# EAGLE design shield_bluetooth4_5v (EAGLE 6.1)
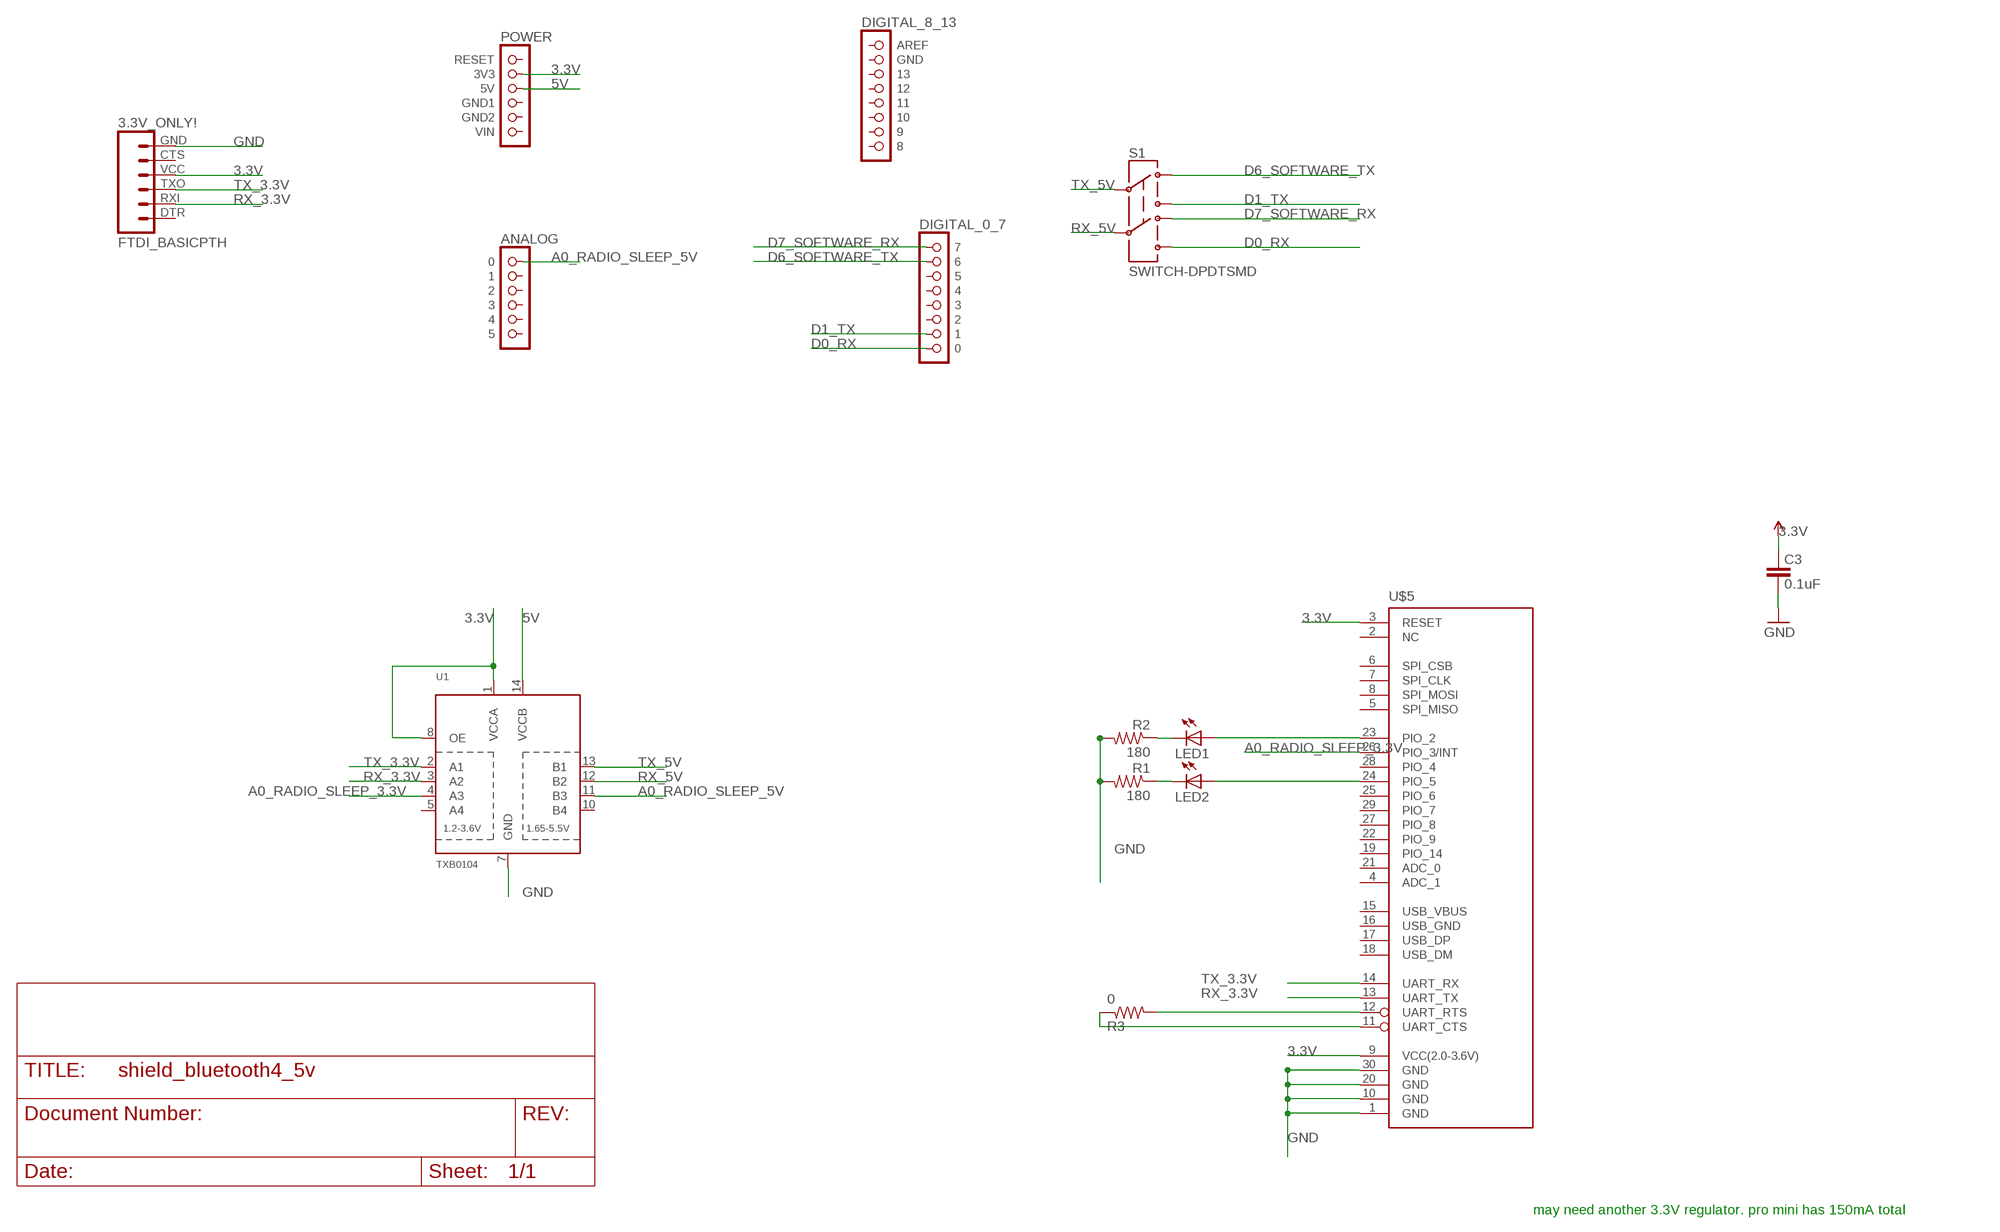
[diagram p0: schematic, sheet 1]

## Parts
3.3V_ONLY!  FTDI_BASICPTH  [FTDI_BASIC]
C3  0.1uF  CAP0402-CAP  [0402-CAP]
LED1  LED0603  [LED-0603]
LED2  LED0603  [LED-0603]
R1  180  RESISTOR0402-RES  [0402-RES]
R2  180  RESISTOR0402-RES  [0402-RES]
R3  0  RESISTOR0402-RES  [0402-RES]
S1  SWITCH-DPDTSMD  [AYZ0202]
U1  TXB0104  TXB0104PWRSOIC14  [SO14]
U$1  POWER  [1X06]
U$2  ANALOG  [1X06]
U$3  DIGITAL_0_7  [1X08]
U$4  DIGITAL_8_13  [1X08]
U$5  BLUERADIO_BR-LE4.0-S2  [BLUERADIO_BR-LE4.0-S2]

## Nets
3.3V: 3.3V_ONLY!.VCC C3.2 U1.1(VCCA) U1.8(OE) U$1.2(3V3) U$5.3(RESET) U$5.9(VCC(2.0-3.6V)) ; supply symbol labelled VCC
5V: U1.14(VCCB) U$1.3(5V)
A0_RADIO_SLEEP_3.3V: U1.4(A3) U$5.26(PIO_3/INT)
A0_RADIO_SLEEP_5V: U1.11(B3) U$2.1
D0_RX: S1.6 U$3.8
D1_TX: S1.3 U$3.7
D6_SOFTWARE_TX: S1.1 U$3.2
D7_SOFTWARE_RX: S1.4 U$3.1
GND [vcc]: 3.3V_ONLY!.GND C3.1 R1.2 R2.2 U1.7(GND) U$5.1(GND) U$5.10(GND) U$5.20(GND) U$5.30(GND)
N$1: LED2.A U$5.24(PIO_5)
N$2: LED1.C R2.1
N$3: LED1.A U$5.23(PIO_2)
N$4: LED2.C R1.1
N$5: R3.2 U$5.12(UART_RTS)
N$9: R3.1 U$5.11(UART_CTS)
RX_3.3V: 3.3V_ONLY!.RXI U1.3(A2) U$5.13(UART_TX)
RX_5V: S1.5 U1.12(B2)
TX_3.3V: 3.3V_ONLY!.TXO U1.2(A1) U$5.14(UART_RX)
TX_5V: S1.2 U1.13(B1)
Unconnected: 3.3V_ONLY!.CTS 3.3V_ONLY!.DTR U1.5(A4) U1.10(B4) U$1.1(RESET) U$1.4(GND1) U$1.5(GND2) U$1.6(VIN) U$2.2 U$2.3 U$2.4 U$2.5 U$2.6 U$3.3 U$3.4 U$3.5 U$3.6 U$4.1(AREF) U$4.2(GND) U$4.3 U$4.4 U$4.5 U$4.6 U$4.7 U$4.8 U$5.2(NC) U$5.4(ADC_1) U$5.5(SPI_MISO) U$5.6(SPI_CSB) U$5.7(SPI_CLK) U$5.8(SPI_MOSI) U$5.15(USB_VBUS) U$5.16(USB_GND) U$5.17(USB_DP) U$5.18(USB_DM) U$5.19(PIO_14) U$5.21(ADC_0) U$5.22(PIO_9) U$5.25(PIO_6) U$5.27(PIO_8) U$5.28(PIO_4) U$5.29(PIO_7)

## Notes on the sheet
- may need another 3.3V regulator. pro mini has 150mA total

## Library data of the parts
3.3V_ONLY! = SparkFun-Connectors:FTDI_BASIC: FTDI Basic header with labels
C3 = SparkFun:CAP: Capacitor
LED1 LED2 = SparkFun-LED:LED: LEDs
R1-R3 = SparkFun-Passives:RESISTOR: Resistor
S1 = SparkFun-Electromechanical:SWITCH-DPDT: DPDT Version of the COM-00597
U1 = adafruit-2012:TXB0104PWR: 4-Bit Bi-Directional Level Shifter 1.2V-3.6V (VCCA) to 1.65V-5.5V (VCCB) bi-directional level shifter with auto direction sensing. Max data rate - VCCA 1.8V: 20Mbps (50ns), VCCA 3.3V: 100Mbps (10ns) Digikey: 296-21929-1-ND
U$1 = arduino:POWER
U$2 = arduino:ANALOG
U$3 = arduino:DIGITAL_0_7
U$4 = arduino:DIGITAL_8_13
U$5 = SparkFun-RF:BLUERADIO_BR-LE4.0-S2

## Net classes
1 vcc: width 0.254 mm

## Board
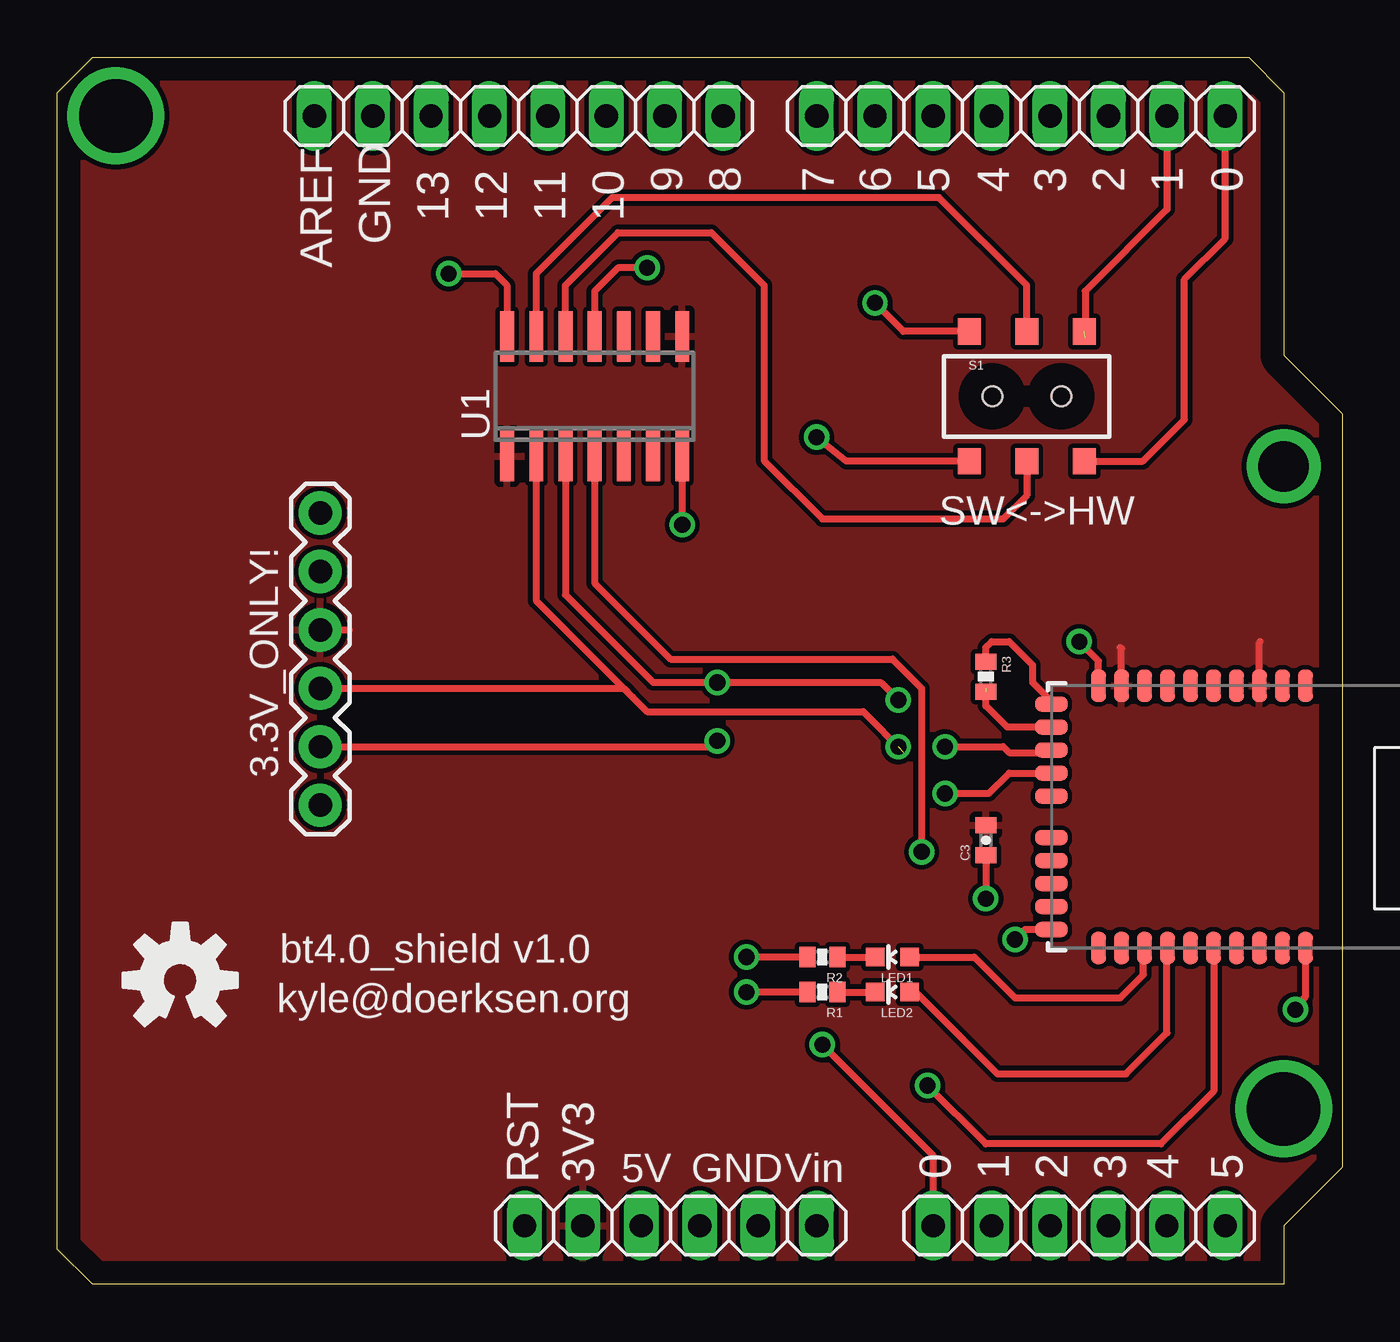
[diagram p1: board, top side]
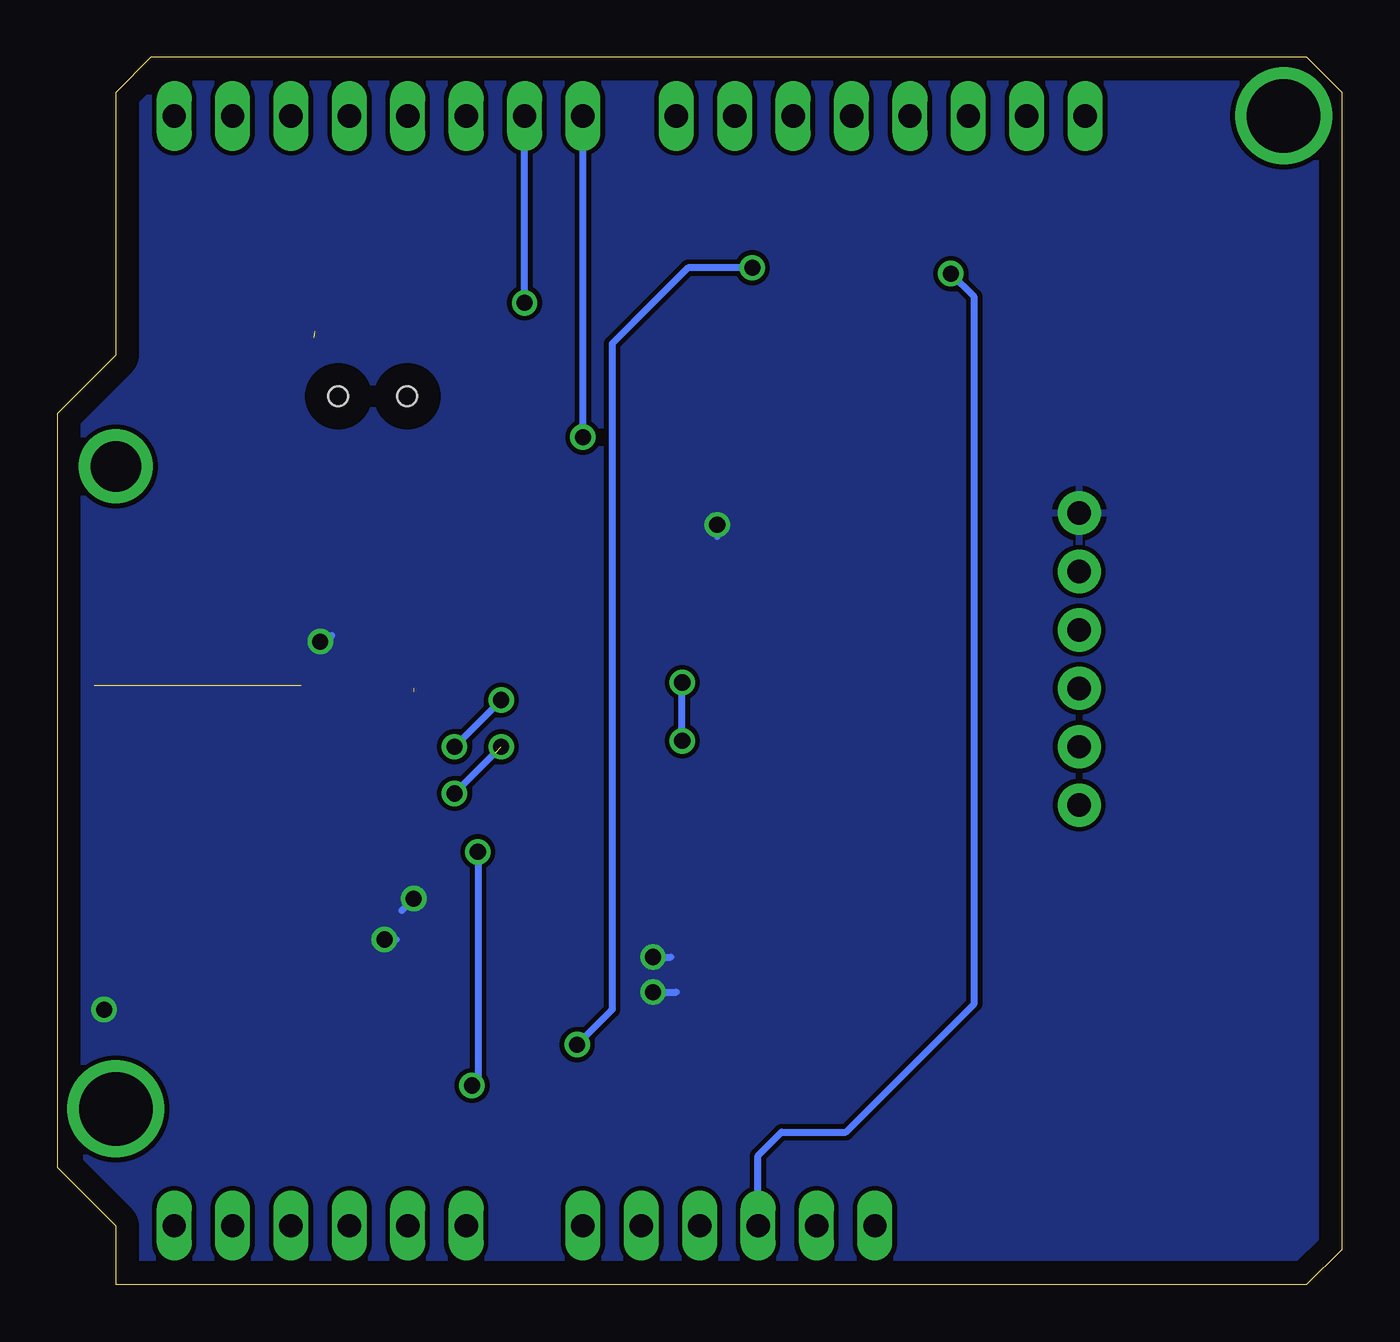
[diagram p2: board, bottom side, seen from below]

Size 55.88 x 53.34 mm. Coordinates in mm from the lower left corner, seen from the top.
Outline: 0,51.82 1.52,53.34 51.82,53.34 53.34,51.82 53.34,40.39 55.88,37.85 55.88,5.08 53.34,2.54 53.34,0 1.52,0 0,1.52 0,51.82
Copper layers (1*16): Top 0.035mm / dielectric 1.5mm / Bottom 0.035mm
Design rules: minimum track width 10mil, minimum drill 24mil, track to track 8mil, track to pad 8mil, pad to pad 8mil, via to via 8mil, smd to smd 8mil, copper to edge 40mil, drill to drill 8mil, minimum pad ring 10mil, minimum via ring 8mil, stop-mask expansion 4mil, vias tented up to drill 0mil, thermal gap 10mil

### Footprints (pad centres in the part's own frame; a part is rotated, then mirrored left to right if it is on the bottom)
FTDI_BASIC = drill 1.016 pad 1.88: CTS 10.16,0; DTR 0,0; GND 12.7,0; RXI 2.54,0; TXO 5.08,0; VCC 7.62,0
0402-CAP = smd 0.7 x 0.9: 1 -0.65,0; 2 0.65,0
LED-0603 = smd 0.8 x 0.8: A 0,-0.75; C 0,0.75
0402-RES = smd 0.7 x 0.9: 1 -0.65,0; 2 0.65,0
AYZ0202 = smd 1 x 1.15: 1 -2.5,2.825; 2 0,2.825; 3 2.5,2.825; 4 -2.5,-2.825; 5 0,-2.825; 6 2.5,-2.825 | hole 0.85: 1.5,0; -1.5,0
SO14 = smd 0.6 x 2.2: 1 -3.81,-2.6; 2 -2.54,-2.6; 3 -1.27,-2.6; 4 0,-2.6; 5 1.27,-2.6; 6 2.54,-2.6; 7 3.81,-2.6; 8 3.81,2.6; 9 2.54,2.6; 10 1.27,2.6; 11 0,2.6; 12 -1.27,2.6; 13 -2.54,2.6; 14 -3.81,2.6
1X06 = drill 1.016 long: 1 -6.35,0; 2 -3.81,0; 3 -1.27,0; 4 1.27,0; 5 3.81,0; 6 6.35,0
1X08 = drill 1.016 long: 1 -8.89,0; 2 -6.35,0; 3 -3.81,0; 4 -1.27,0; 5 1.27,0; 6 3.81,0; 7 6.35,0; 8 8.89,0
BLUERADIO_BR-LE4.0-S2 = smd 0.65 x 1.4: 1 -4.5,-5.7; 2 -3.5,-5.7; 3 -2.5,-5.7; 4 -1.5,-5.7; 5 -0.5,-5.7; 6 0.5,-5.7; 7 1.5,-5.7; 8 2.5,-5.7; 9 3.5,-5.7; 10 4.5,-5.7; 21 4.5,5.7; 22 3.5,5.7; 23 2.5,5.7; 24 1.5,5.7; 25 0.5,5.7; 26 -0.5,5.7; 27 -1.5,5.7; 28 -2.5,5.7; 29 -3.5,5.7; 30 -4.5,5.7 | smd 1.4 x 0.65: 11 6.55,-4.9; 12 6.55,-3.9; 13 6.55,-2.9; 14 6.55,-1.9; 15 6.55,-0.9; 16 6.55,0.9; 17 6.55,1.9; 18 6.55,2.9; 19 6.55,3.9; 20 6.55,4.9

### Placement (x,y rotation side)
3.3V_ONLY!  11.43,20.83 90 top
C3  40.39,19.3 90 top
LED1  36.32,14.22 90 top
LED2  36.32,12.7 90 top
R1  33.27,12.7 180 top
R2  33.27,14.22 180 top
R3  40.39,26.42 270 top
S1  42.16,38.61 0 top
U1  23.37,38.61 0 top
U$1  26.67,2.54 0 top
U$2  44.45,2.54 0 top
U$3  41.91,50.8 0 top
U$4  20.07,50.8 0 top
U$5  49.78,20.32 180 top
U$7  [OSHW-LOGO-M]  5.33,13.21 0 top

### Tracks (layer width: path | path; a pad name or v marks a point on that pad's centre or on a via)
3.3V
  Top 0.305: 3.3V_ONLY!.VCC 12.7,28.45 | U$5.9 46.28,27.63 46.23,27.69 | U$5.3 52.28,27.9 52.32,27.94
  pour Top: 0,56.13 -0.25,56.13 -0.25,-7.87 71.63,-7.87 71.63,54.86 1.02,54.86 1.02,56.13
5V  (via drill 0.7)
  Top 0.305: v17.02,43.94 19.05,43.94 19.56,43.43 U1.14
  Bottom 0.305: U$1.3 25.4,5.59 24.38,6.6 21.59,6.6 16,12.19 16,42.93 v17.02,43.94
A0_RADIO_SLEEP_3.3V  (via drill 0.7)
  Top 0.305: U1.4 23.37,30.48 26.67,27.18 36.32,27.18 37.59,25.91 v37.59,18.8 | U$5.26 50.29,14.61 50.29,8.38 48.01,6.1 40.39,6.1 v37.85,8.64
  Bottom 0.305: v37.59,18.8 37.59,8.89 v37.85,8.64
A0_RADIO_SLEEP_5V  (via drill 0.7)
  Top 0.305: U$2.1 38.1,5.59 v33.27,10.41 | v25.65,44.2 24.38,44.2 23.37,43.18 U1.11
  Bottom 0.305: v25.65,44.2 28.45,44.2 31.75,40.89 31.75,11.94 v33.27,10.41
D0_RX
  Top 0.305: S1.6 47.21,35.78 49.02,37.59 49.02,43.69 50.8,45.47 U$3.8
D1_TX  (1 unrouted)
  Top 0.305: U$3.7 48.26,46.74 44.7,43.18 44.7,41.15
D6_SOFTWARE_TX  (via drill 0.7)
  Top 0.305: S1.1 36.8,41.43 v35.56,42.67
  Bottom 0.305: v35.56,42.67 U$3.2
D7_SOFTWARE_RX  (via drill 0.7)
  Top 0.305: S1.4 34.32,35.78 v33.02,36.83
  Bottom 0.305: v33.02,36.83 U$3.1
GND  (via drill 0.7)  (1 unrouted)
  Top 0.305: C3.1 v40.39,16.76 | U$5.20 42.09,15.42 v41.66,14.99 | U$5.30 54.28,12.52 v53.85,11.94 | R2.2 v29.97,14.22 | R1.2 v29.97,12.7 | U1.7 27.18,33.53 v27.18,33.02 | U$5.10 45.28,27.11 v44.45,27.94
  Bottom 0.305: v40.39,16.76 40.89,16.26 | v41.66,14.99 41.15,14.99 | v53.85,11.94 53.59,12.19 | v29.97,14.22 29.21,14.22 | v29.97,12.7 28.96,12.7 | v27.18,33.02 27.18,32.51 | v44.45,27.94 44.2,27.94 43.94,28.19
  pour Bottom: -1.52,58.42 74.42,58.42 74.42,-10.41 -1.52,-10.41
N$1
  Top 0.305: LED2.A 37.34,12.7 40.89,9.14 46.48,9.14 48.26,10.92 48.26,14.6 U$5.24
N$2
  Top 0.305: R2.1 LED1.C
N$3
  Top 0.305: LED1.A 39.88,14.22 41.66,12.45 46.23,12.45 47.24,13.46 47.24,14.58 U$5.23
N$4
  Top 0.305: R1.1 LED2.C
N$5  (1 unrouted)
  Top 0.305: U$5.12 41.31,24.22 40.39,25.15 40.39,25.91
N$6  (via drill 3.2)
  other vias: 2.54,50.8
N$7  (via drill 3.2)
  other vias: 53.34,7.62
N$8  (via drill 2.2)
  other vias: 53.34,35.56
N$9
  Top 0.305: U$5.11 43.23,25.35 42.93,25.65 42.42,26.16 42.42,26.92 41.4,27.94 40.64,27.94 40.39,27.69 R3.1
RX_3.3V  (via drill 0.7)
  Top 0.305: U1.3 22.1,29.97 25.91,26.16 v28.7,26.16 | v28.7,26.16 30.23,26.16 | 3.3V_ONLY!.RXI 28.45,23.37 v28.7,23.62 | v38.61,23.37 41.15,23.37 41.4,23.11 43.13,23.11 U$5.13 | 35.81,26.16 v36.58,25.4 35.81,26.16 | v28.7,26.16 35.81,26.16
  Bottom 0.305: v36.58,25.4 v38.61,23.37 | v28.7,23.62 28.7,25.65 v28.7,26.16
RX_5V
  Top 0.305: S1.5 42.16,34.29 41.15,33.27 33.27,33.27 30.73,35.81 30.73,43.43 28.45,45.72 24.38,45.72 22.1,43.43 U1.12
TX_3.3V  (via drill 0.7)  (1 unrouted)
  Top 0.305: U1.2 20.83,29.72 25.02,25.53 | 25.02,25.53 25.65,24.89 35.05,24.89 36.83,23.11 | 43.11,22.1 U$5.14 41.4,22.23 40.51,21.34 v38.61,21.34 | 3.3V_ONLY!.TXO 24.64,25.91 25.02,25.53
  Bottom 0.305: v36.58,23.37 v38.61,21.34
TX_5V
  Top 0.305: S1.2 42.16,43.43 38.35,47.24 24.13,47.24 20.83,43.94 U1.13

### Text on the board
tPlace: SW<->HW | bt4.0_shield v1.0 | kyle@doerksen.org
tNames: 9 | 8 | 7 | 6 | 5 | 4 | 3 | 2 | 1 | 0 | 13 | 12 | 11 | 10 | GND | AREF | 0 | 1 | 2 | 3 | 4 | 5 | RST | 3V3 | 5V | GND | Vin
TallParts: USB | ISP | PWR
ArduinoHoles: 3.2mm | 2.2mm | 3.2mm

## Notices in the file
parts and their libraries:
SparkFun-RF: Licensing: CC v3.0 Share-Alike You are welcome to use this library for commercial purposes.
